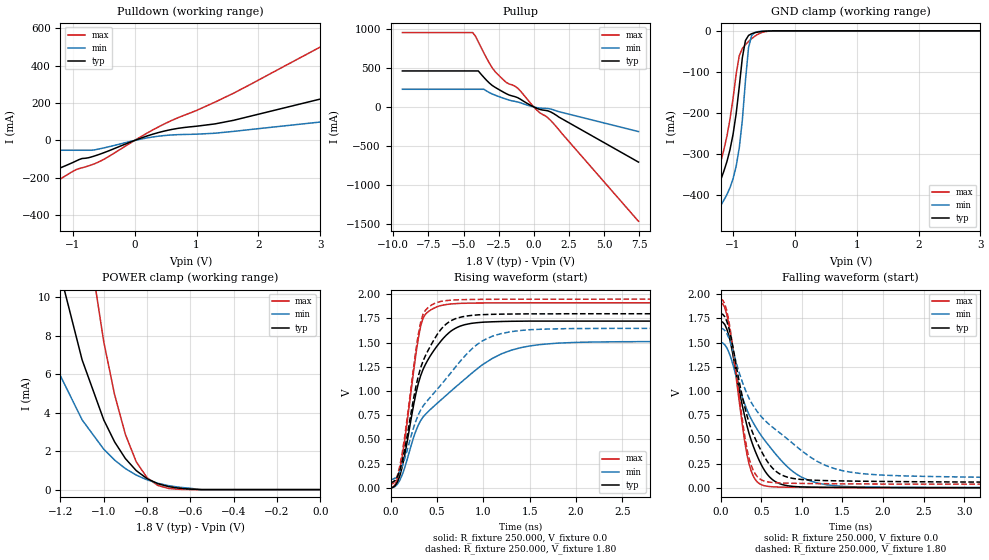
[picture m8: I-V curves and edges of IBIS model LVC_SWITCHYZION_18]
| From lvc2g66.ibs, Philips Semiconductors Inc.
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|   Model LVC_SWITCHYZION_18
[Model]   LVC_SWITCHYZION_18
Model_type   I/O
Polarity   Non-Inverting
Enable   Active-High
Vinl  =  0.63V
Vinh  =  1.17V
Vmeas =  0.90V
Cref  =  30.0pF
Rref  =  1.0k
Vref  =  0.0V
C_comp   8.21pF   4.64pF   10.52pF
[Model Spec]
| Note: The input and output voltage ratings may be exceeded if the input and
|   output current ratings are observed (please refer to the data sheet)
|   Subparameter   typ   min   max
| Thresholds
Vinh   1.17   1.0725   1.2675
Vinl   0.63   0.5775   0.6825
| Overshoot
S_overshoot_high   6.5   6.5   6.5   | Static overshoot
S_overshoot_low   -0.5   -0.5   -0.5
D_overshoot_high   7.2   7.2   7.2   | Dynamic overshoot
D_overshoot_low   -0.95   -0.9   -1.0
D_overshoot_time   3n   3n   3n
| Timing Thresholds
Vmeas   0.9   0.825   0.975
|Ambient temperature:   25   85   -40
[Temperature Range]   25   85   -40
[Voltage Range]   1.80V   1.65V   1.95V
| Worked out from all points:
|   slope of the pulldown table from 0 to 0.27 V, typ, clamps not added: 8.71 ohm
|   slope of the pullup table from 0 to 0.27 V, typ, clamps not added: 12.5 ohm
|   GND clamp passes 1 mA (typ) near -0.49 V on its own axis
|   POWER clamp passes 1 mA (typ) near -0.85 V on its own axis
|   rising waveform, R_fixture 250.000, V_fixture 0.0: 20-80 % time 283ps typ, 726ps min, 161ps max; typ from 0 V to 1.72 V
|   rising waveform, R_fixture 250.000, V_fixture 1.80: 20-80 % time 268ps typ, 594ps min, 161ps max; typ from 0.056 V to 1.8 V
|   falling waveform, R_fixture 250.000, V_fixture 0.0: 20-80 % time 292ps typ, 553ps min, 186ps max; typ from 1.72 V to 0 V
|   falling waveform, R_fixture 250.000, V_fixture 1.80: 20-80 % time 334ps typ, 794ps min, 190ps max; typ from 1.8 V to 0.056 V
|Process Range   nominal   slow   fast
[Pulldown]
| voltage   I(typ)   I(min)   I(max)
-5.5V     -269.6mA   -52.48mA   -458.5mA
-2.3V     -269.6mA   -52.48mA   -458.5mA
-2.1V     -269.6mA   -52.48mA   -399.9mA
-1.7V     -212.1mA   -52.48mA   -307.2mA
-1V       -118mA     -52.48mA   -165.3mA
-700mV    -88.3mA    -52.48mA   -131mA
400mV     43.47mA    23.26mA    74.9mA
1.6V      107.6mA    48.36mA    252.5mA
3.4V      253.4mA    112.4mA    569.6mA
3.7V      277.7mA    123mA      622.5mA
7.6V      593.7mA    261mA      1.311A
11V       869.2mA    381.2mA    1.91A
[Pullup]
| voltage   I(typ)   I(min)   I(max)
-9.35V    460.4mA    225.7mA    951.6mA
-4.35V    460.4mA    225.7mA    951.6mA
-4.15V    460.4mA    225.7mA    905.6mA
-3.95V    460.4mA    225.7mA    834mA
-3.55V    377.3mA    225.7mA    690.4mA
-3.15V    303.5mA    181.6mA    556.5mA
-2.75V    250.5mA    150.1mA    451.1mA
-1.95V    168.5mA    98.33mA    312.2mA
-1.15V    118.7mA    63.25mA    240.4mA
200mV     -16.62mA   -8.053mA   -37.82mA
1.2V      -64.27mA   -26.68mA   -173.1mA
7.45V     -706.5mA   -315.6mA   -1.464A
[GND_clamp]
| voltage   I(typ)   I(min)   I(max)
-5.5V     -5.559A    -5.191A    -6.237A
-1.4V     -516.8mA   -571.9mA   -482.3mA
-1.35V    -470.4mA   -526mA     -435.3mA
-1.3V     -426.1mA   -482.4mA   -389.9mA
-1.1V     -319.6mA   -399.9mA   -257.5mA
-950mV    -202.3mA   -330.6mA   -105.9mA
-900mV    -136.6mA   -286mA     -60.85mA
-850mV    -65.6mA    -218.1mA   -43.04mA
-800mV    -23.77mA   -122.2mA   -33.79mA
-750mV    -11.27mA   -41.07mA   -26.09mA
-650mV    -4.723mA   -4.118mA   -13.33mA
5.5V      416.7pA    5.546nA    31.12pA
[POWER_clamp]
| voltage   I(typ)   I(min)   I(max)
-9.35V    7.563A     7.588A     7.617A
-1.4V     22.06mA    13.37mA    49.16mA
-1.25V    13.4mA     7.056mA    30.15mA
-1.1V     6.748mA    3.627mA    15.04mA
-1V       3.626mA    2.101mA    7.687mA
-950mV    2.484mA    1.537mA    4.945mA
-900mV    1.614mA    1.093mA    2.868mA
-850mV    989.1uA    756.2uA    1.451mA
-800mV    571.3uA    508.4uA    620uA
-750mV    308uA      329uA      214.1uA
-650mV    69.74uA    122uA      13.79uA
0V        0A         0A         0A
[Ramp]
| variable   typ   min   max
dV/dt_r   1.033V/283.479ps   907.138mV/725.812ps   1.147V/161.120ps
dV/dt_f   1.047V/333.646ps   936.469mV/793.498ps   1.147V/189.673ps
R_load = 250.000
[Rising Waveform]
R_fixture   = 250.000
V_fixture   = 0.0
V_fixture_min = 0.0
V_fixture_max = 0.0
| time   V(typ)   V(min)   V(max)
0s        99.81fV    5.526pV    16.79fV
75ps      61.8mV     39.75mV    94.13mV
125ps     214.1mV    133.5mV    317.1mV
325ps     1.161V     696.3mV    1.674V
375ps     1.274V     758.2mV    1.793V
550ps     1.525V     914mV      1.885V
750ps     1.671V     1.082V     1.906V
1.1ns     1.716V     1.339V     1.911V
1.7ns     1.723V     1.488V     1.912V
8.8ns     1.721V     1.512V     1.911V
[Rising Waveform]
R_fixture   = 250.000
V_fixture   = 1.80
V_fixture_min = 1.65
V_fixture_max = 1.95
| time   V(typ)   V(min)   V(max)
0s        55.63mV    86.4mV     38.05mV
50ps      78.71mV    102mV      72.95mV
100ps     182.5mV    166.8mV    227.9mV
275ps     1.056V     697.4mV    1.438V
325ps     1.243V     805.8mV    1.714V
400ps     1.412V     904.6mV    1.859V
550ps     1.646V     1.072V     1.928V
1ns       1.79V      1.524V     1.948V
1.5ns     1.798V     1.634V     1.949V
8.8ns     1.8V       1.649V     1.95V
[Falling Waveform]
R_fixture   = 250.000
V_fixture   = 0.0
V_fixture_min = 0.0
V_fixture_max = 0.0
| time   V(typ)   V(min)   V(max)
0s        1.719V     1.502V     1.911V
100ps     1.574V     1.403V     1.689V
275ps     816.6mV    915mV      599.6mV
350ps     560mV      755.1mV    245.1mV
425ps     379.3mV    637.7mV    86.85mV
525ps     201mV      510.7mV    25.15mV
700ps     52.63mV    326.4mV    8.795mV
975ps     10.6mV     120.8mV    5.187mV
1.5ns     4.837mV    16mV       2.448mV
8.8ns     33.56uV    569.2uV    124nV
[Falling Waveform]
R_fixture   = 250.000
V_fixture   = 1.80
V_fixture_min = 1.65
V_fixture_max = 1.95
| time   V(typ)   V(min)   V(max)
0s        1.8V       1.65V      1.95V
100ps     1.654V     1.55V      1.728V
275ps     912.2mV    1.075V     654.6mV
350ps     669.7mV    924.2mV    302.5mV
425ps     508.6mV    818.4mV    145.3mV
550ps     305.6mV    692.1mV    67.05mV
850ps     104.5mV    485.5mV    47.97mV
1.3ns     74.92mV    229mV      42.77mV
1.8ns     67.97mV    142.6mV    40.23mV
8.8ns     55.7mV     89.22mV    38.05mV
